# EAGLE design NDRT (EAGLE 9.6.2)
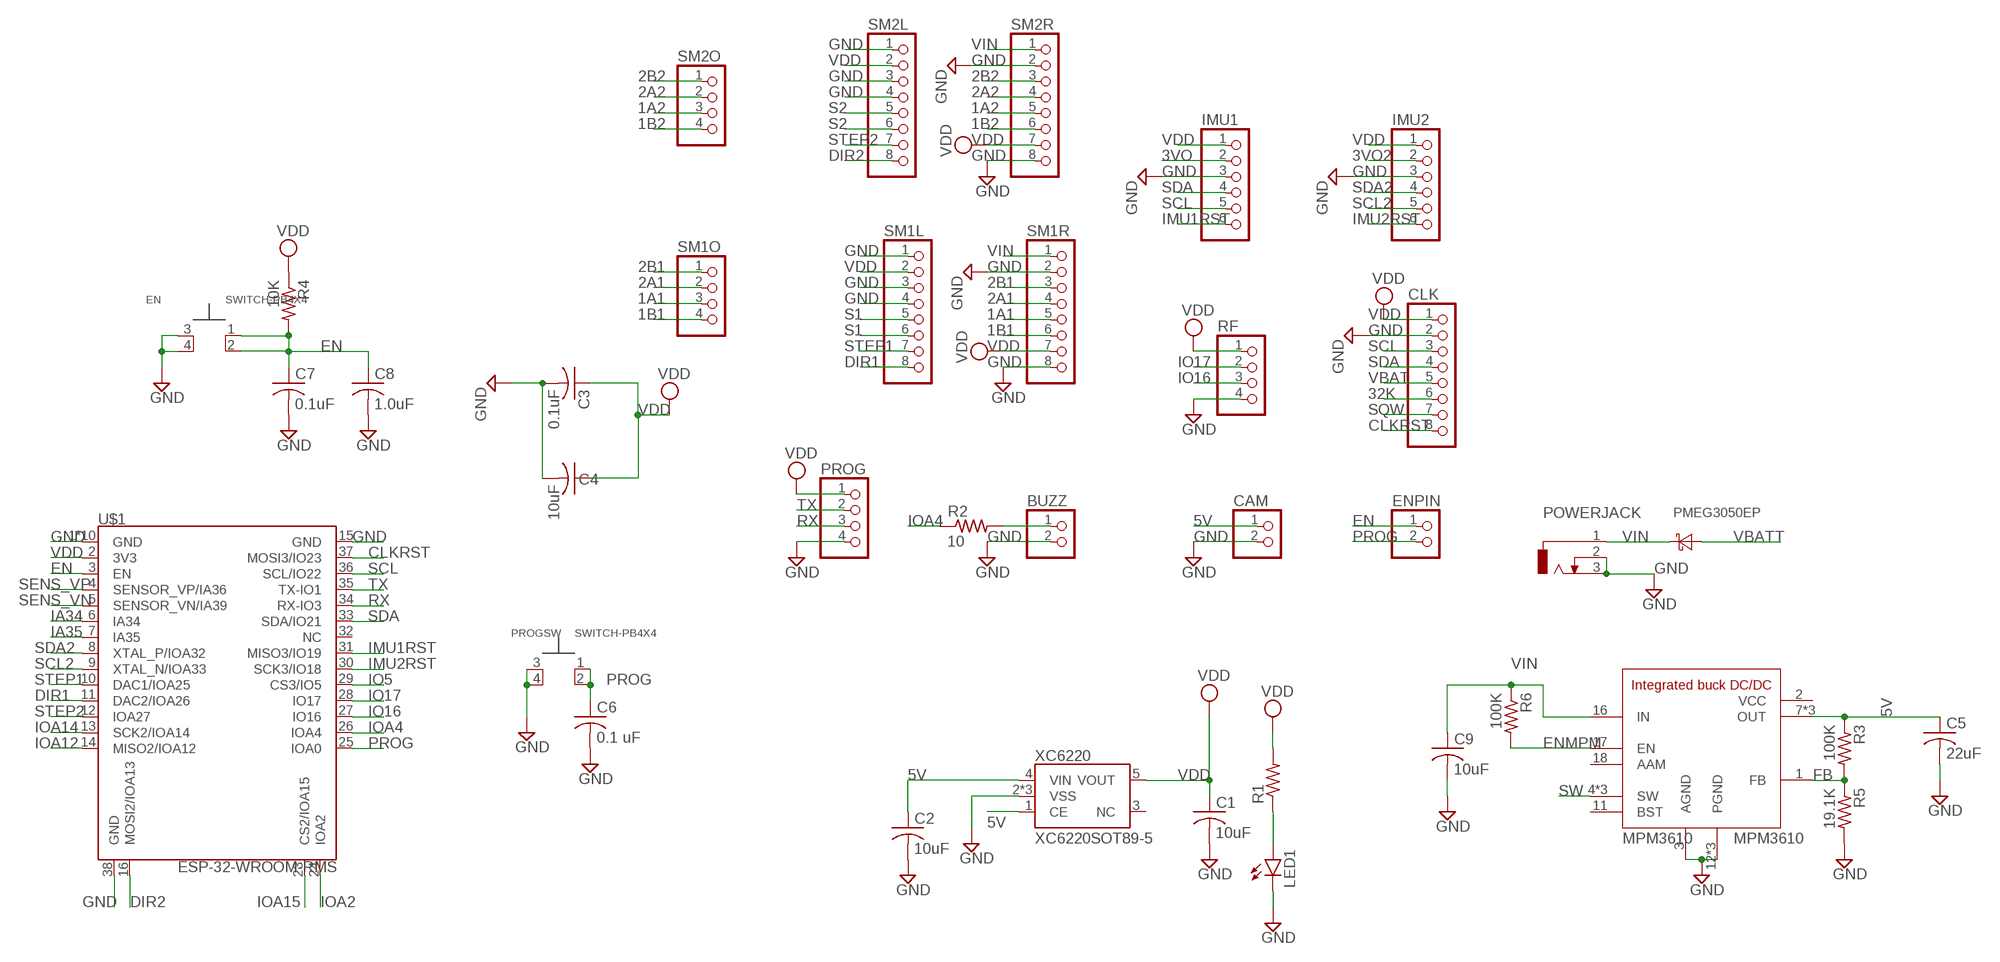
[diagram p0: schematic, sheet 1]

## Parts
BUZZ  PINHD-1X2S  [1X02N]
C1  10uF  C-USC0805  [C0805]
C2  10uF  C-USC0805  [C0805]
C3  0.1uF  C-USC0603  [C0603]
C4  10uF  C-USC0805  [C0805]
C5  22uF  C-USC0805  [C0805]
C6  0.1 uF  C-USC0603  [C0603]
C7  0.1uF  C-USC0603  [C0603]
C8  1.0uF  C-USC0603  [C0603]
C9  10uF  C-USC0805  [C0805]
CAM  PINHD-1X2S  [1X02N]
CLK  PINHD-1X8  [1X08]
EN  SWITCH-PB4X4  [PBSMT4X4M]
ENPIN  PINHD-1X2S  [1X02N]
IMU1  PINHD-1X6  [1X06]
IMU2  PINHD-1X6  [1X06]
LED1  LEDCHIPLED_0603  [CHIPLED_0603]
MPM3610  MICROBUILDER_MPM3610  [MICROBUILDER_MPM3610]
PMEG3050EP  DIODE-SCHOTTKY-SOD128  [SOD128]
POWERJACK  DCJ0303  [DCJ0303]
PROG  PINHD-1X4  [1X04N]
PROGSW  SWITCH-PB4X4  [PBSMT4X4M]
R1  R-US_R0603  [R0603]
R2  10  R-US_R0603  [R0603]
R3  100K  R-US_R0603  [R0603]
R4  10K  R-US_R0603  [R0603]
R5  19.1K  R-US_R0603  [R0603]
R6  100K  R-US_R0603  [R0603]
RF  PINHD-1X4  [1X04N]
SM1L  PINHD-1X8  [1X08]
SM1O  PINHD-1X4  [1X04N]
SM1R  PINHD-1X8  [1X08]
SM2L  PINHD-1X8  [1X08]
SM2O  PINHD-1X4  [1X04N]
SM2R  PINHD-1X8  [1X08]
U$1  ESP-32-WROOM-RMS  [ESP-WROOM-32D]
XC6220  XC6220SOT89-5  [SOT89-5]

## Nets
1A1: SM1O.3 SM1R.5
1A2: SM2O.3 SM2R.5
1B1: SM1O.4 SM1R.6
1B2: SM2O.4 SM2R.6
2A1: SM1O.2 SM1R.4
2A2: SM2O.2 SM2R.4
2B1: SM1O.1 SM1R.3
2B2: SM2O.1 SM2R.3
3VO [not power]: IMU1.2
3VO2 [not power]: IMU2.2
5V: C2.1 C5.1 CAM.1 MPM3610.7(OUT) MPM3610.8(OUT) MPM3610.9(OUT) R3.1 XC6220.1(CE) XC6220.4(VIN)
32K [not power]: CLK.6
CLKRST: CLK.8 U$1.37(MOSI3/IO23)
DIR1: SM1L.8 U$1.11(DAC2/IOA26)
DIR2: SM2L.8 U$1.16(MOSI2/IOA13)
EN: C7.1 C8.1 EN.1 EN.2 ENPIN.1 R4.2 U$1.3(EN)
ENMPM: MPM3610.17(EN) R6.2
FB: MPM3610.1(FB) R3.2 R5.1
GND: BUZZ.2 C1.2 C2.2 C3.2 C4.2 C5.2 C6.2 C7.2 C8.2 C9.2 CAM.2 CLK.2 EN.3 EN.4 IMU1.3 IMU2.3 LED1.C MPM3610.3(AGND) MPM3610.12(PGND) MPM3610.13(PGND) MPM3610.14(PGND) POWERJACK.2 POWERJACK.3 PROG.4 PROGSW.3 PROGSW.4 R5.2 RF.4 SM1L.1 SM1L.3 SM1L.4 SM1R.2 SM1R.8 SM2L.1 SM2L.3 SM2L.4 SM2R.2 SM2R.8 U$1.1(GND) U$1.15(GND) U$1.38(GND) U$1.GND U$1.GNDT1(GND) U$1.GNDT2(GND) U$1.GNDT3(GND) U$1.GNDT4(GND) U$1.GNDT5(GND) U$1.GNDT6(GND) U$1.GNDT7(GND) U$1.GNDT8(GND) XC6220.2(VSS) XC6220.6(VSS) XC6220.7(VSS)
IA34 [not power]: U$1.6(IA34)
IA35 [not power]: U$1.7(IA35)
IMU1RST: IMU1.6 U$1.31(MISO3/IO19)
IMU2RST: IMU2.6 U$1.30(SCK3/IO18)
IO5 [not power]: U$1.29(CS3/IO5)
IO16: RF.3 U$1.27(IO16)
IO17: RF.2 U$1.28(IO17)
IOA2 [not power]: U$1.24(IOA2)
IOA4: R2.1 U$1.26(IOA4)
IOA12 [not power]: U$1.14(MISO2/IOA12)
IOA14 [not power]: U$1.13(SCK2/IOA14)
IOA15 [not power]: U$1.23(CS2/IOA15)
N$1: BUZZ.1 R2.2
N$2: LED1.A R1.1
PROG: C6.1 ENPIN.2 PROGSW.1 PROGSW.2 U$1.25(IOA0)
RX: PROG.3 U$1.34(RX-IO3)
S1: SM1L.5 SM1L.6
S2: SM2L.5 SM2L.6
SCL: CLK.3 IMU1.5 U$1.36(SCL/IO22)
SCL2: IMU2.5 U$1.9(XTAL_N/IOA33)
SDA: CLK.4 IMU1.4 U$1.33(SDA/IO21)
SDA2: IMU2.4 U$1.8(XTAL_P/IOA32)
SENS_VN [not power]: U$1.5(SENSOR_VN/IA39)
SENS_VP [not power]: U$1.4(SENSOR_VP/IA36)
SQW [not power]: CLK.7
STEP1: SM1L.7 U$1.10(DAC1/IOA25)
STEP2: SM2L.7 U$1.12(IOA27)
SW: MPM3610.4(SW) MPM3610.5(SW) MPM3610.6(SW)
TX: PROG.2 U$1.35(TX-IO1)
VBAT [not power]: CLK.5
VBATT: PMEG3050EP.A
VDD: C1.1 C3.1 C4.1 CLK.1 IMU1.1 IMU2.1 PROG.1 R1.2 R4.1 RF.1 SM1L.2 SM1R.7 SM2L.2 SM2R.7 U$1.2(3V3) XC6220.5(VOUT)
VIN: C9.1 MPM3610.16(IN) PMEG3050EP.C POWERJACK.1 R6.1 SM1R.1 SM2R.1
Unconnected: MPM3610.11(BST) MPM3610.18(AAM) U$1.32(NC) XC6220.3(NC)

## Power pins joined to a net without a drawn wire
VCC: MPM3610.2(VCC)

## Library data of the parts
BUZZ CAM ENPIN = newSDlib:PINHD-1X2S: PIN HEADER
C1-C9 = rcl:C-US: CAPACITOR, American symbol; SPICEPREFIX: C
CLK SM1L SM1R SM2L SM2R = pinhead:PINHD-1X8: PIN HEADER
EN PROGSW = newSDlib:SWITCH-PB
IMU1 IMU2 = pinhead:PINHD-1X6: PIN HEADER
LED1 = led:LED: LED
MPM3610 = NDRT:MICROBUILDER_MPM3610
PMEG3050EP = diode:DIODE-SCHOTTKY-: SCHOTTKY DIODE
POWERJACK = con-jack:DCJ0303: DC POWER JACK Source: DCJ0303.pdf; OC_FARNELL: unknown; OC_NEWARK: unknown
PROG RF SM1O SM2O = newSDlib:PINHD-1X4: PIN HEADER
R1-R6 = rcl:R-US_: RESISTOR, American symbol; SPICEPREFIX: R
U$1 = newSDlib:ESP-32-WROOM-RMS
XC6220 = newSDlib:XC6220: Linear Voltage Regulator 1 A max

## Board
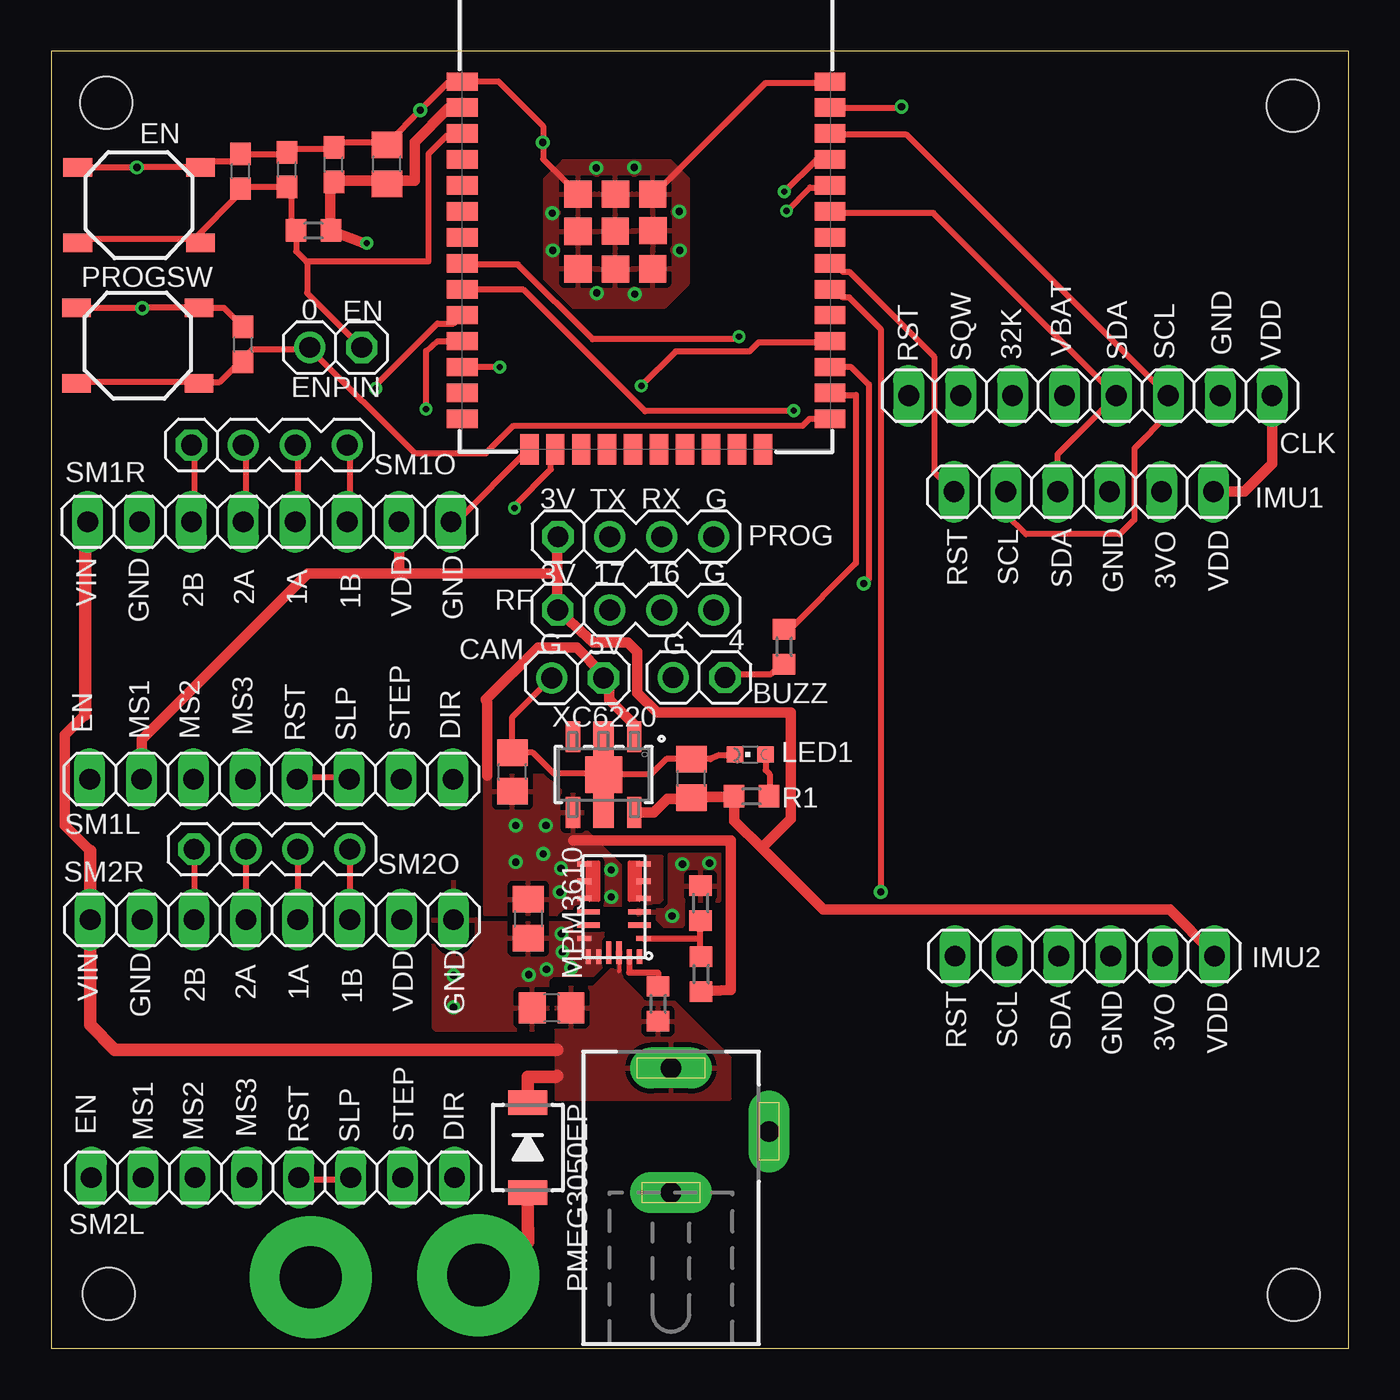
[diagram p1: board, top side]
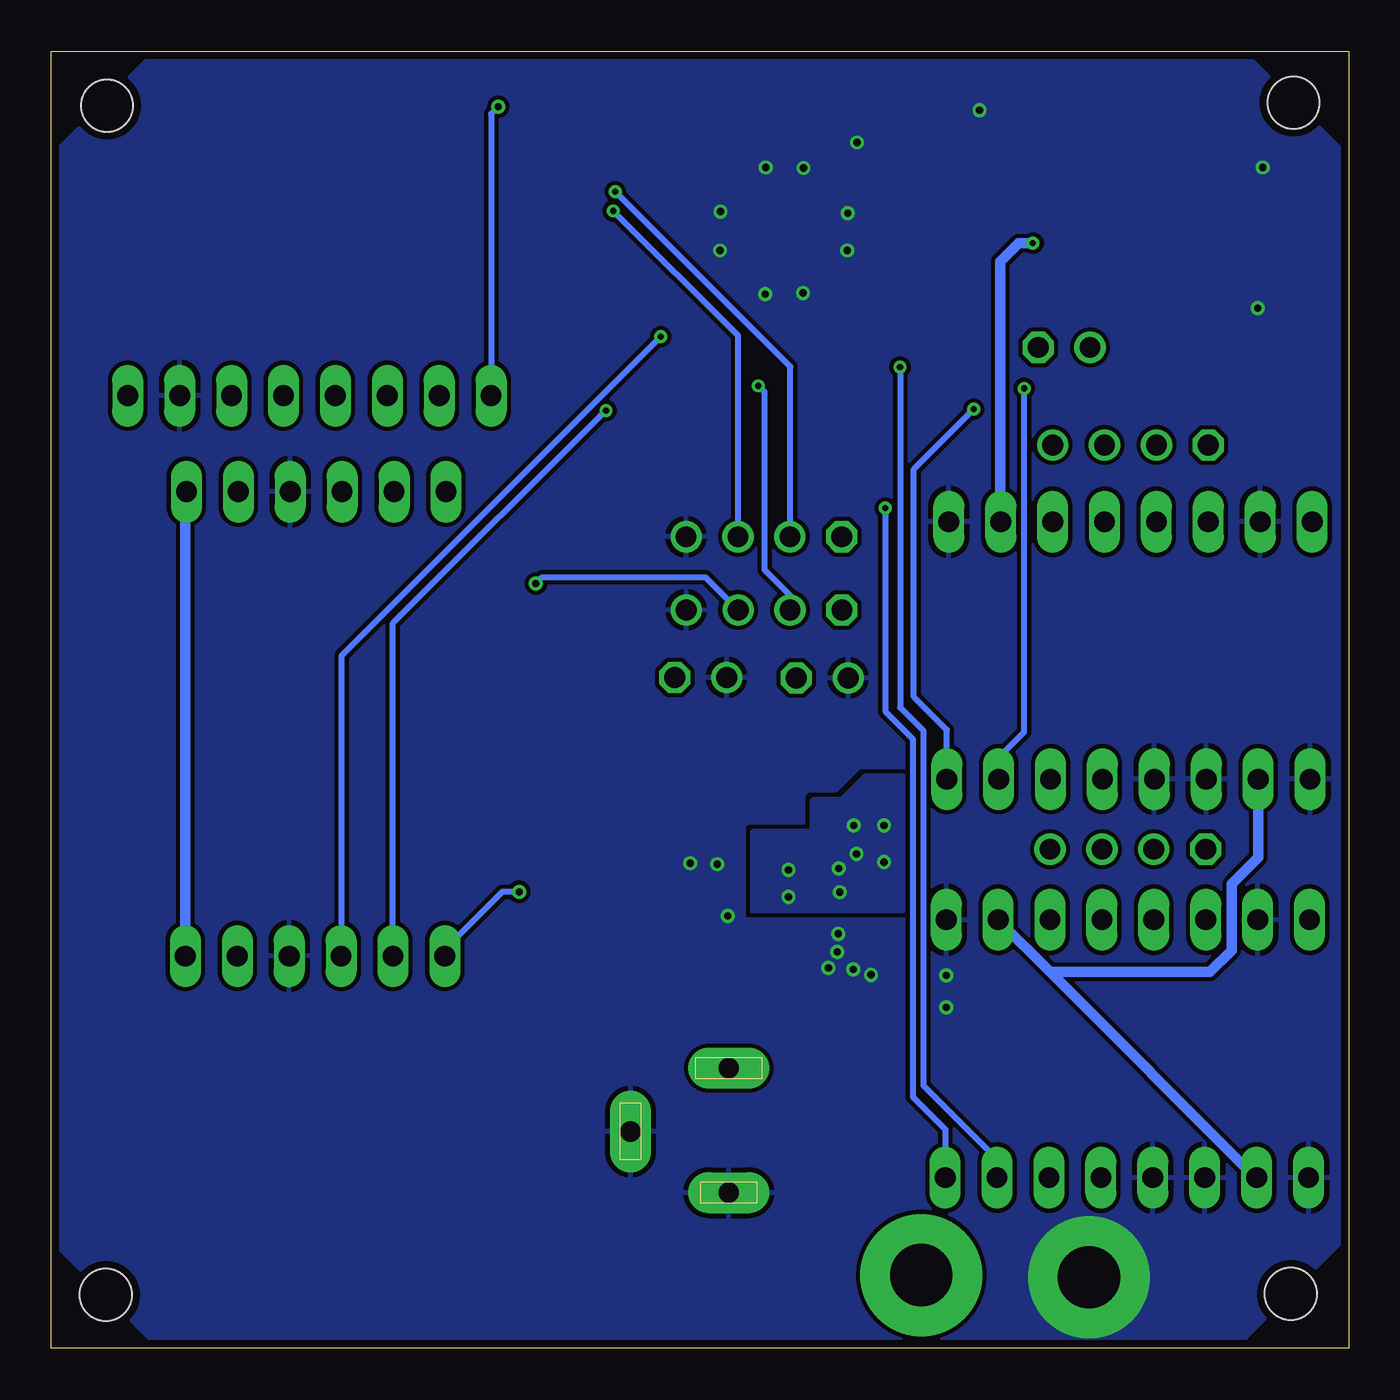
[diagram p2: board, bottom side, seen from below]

Size 63.5 x 63.51 mm. Coordinates in mm from the lower left corner, seen from the top.
Outline: 0,0 63.5,0 63.5,63.51 0.01,63.5 0,0
Copper layers (1*16): Top 0.035559375mm / dielectric 1.6mm / Bottom 0.035559375mm
Design rules "low-cost-2layer": minimum track width 8mil, minimum drill 0.3mm, track to track 8mil, track to pad 8mil, pad to pad 8mil, via to via 8mil, smd to smd 8mil, copper to edge 15mil, drill to drill 8mil, minimum pad ring 6.5mil, minimum via ring 6.5mil, stop-mask expansion 2.5mil, vias tented up to drill 0mil, thermal gap 10mil
Holes 2.54 mm at 2.7,60.99 2.83,2.67 60.82,2.62 60.77,60.84

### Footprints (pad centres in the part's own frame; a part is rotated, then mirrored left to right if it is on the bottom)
1X02N = drill 1.016 octagon: 1 -1.27,0 | drill 1.016: 2 1.27,0
C0805 = smd 1.3 x 1.5: 1 -0.95,0; 2 0.95,0
C0603 = smd 1.1 x 1: 1 -0.85,0; 2 0.85,0
1X08 = drill 1.016 long: 1 -8.89,0; 2 -6.35,0; 3 -3.81,0; 4 -1.27,0; 5 1.27,0; 6 3.81,0; 7 6.35,0; 8 8.89,0
PBSMT4X4M = smd 1.4 x 0.9: 1 -3,1.85; 2 3,1.85; 3 3,-1.85; 4 -3,-1.85
1X06 = drill 1.016 long: 1 -6.35,0; 2 -3.81,0; 3 -1.27,0; 4 1.27,0; 5 3.81,0; 6 6.35,0
CHIPLED_0603 = smd 0.8 x 0.8: A 0,-0.75; C 0,0.75
MICROBUILDER_MPM3610 = smd 0.7 x 0.25: 1 -1.45,1.55; 4 -1.45,-0.4; 5 -1.45,-1.25; 6 -1.45,-2.1; 7 1.45,-2.1; 8 1.45,-1.25; 9 1.45,-0.4; 12 1.45,1.55 | smd 1.1 x 0.25: 2 -1.25,0.9; 3 -1.25,0.25; 10 1.25,0.25; 11 1.25,0.9 | smd 0.25 x 0.7: 13 1.25,2.45; 14 0.75,2.45; 17 -0.75,2.45; 18 -1.25,2.45 | smd 0.25 x 1.1: 15 0.25,2.25; 16 -0.25,2.25
SOD128 = smd 1.2 x 1.9: A 2.2,0; C -2.2,0
DCJ0303 = drill 1 pad 2 long: 1 0,3.1; 2 4.8,0; 3 0,-3
1X04N = drill 1.016 octagon: 1 -3.81,0 | drill 1.016: 2 -1.27,0; 3 1.27,0; 4 3.81,0
R0603 = smd 1 x 1.1: 1 -0.85,0; 2 0.85,0
ESP-WROOM-32D = smd 0.9 x 1.5: 1 7.7,9; 2 6.43,9; 3 5.16,9; 4 3.89,9; 5 2.62,9; 6 1.35,9; 7 0.08,9; 8 -1.19,9; 9 -2.46,9; 10 -3.73,9; 11 -5,9; 12 -6.27,9; 13 -7.54,9; 14 -8.81,9; 25 -8.81,-9; 26 -7.54,-9; 27 -6.27,-9; 28 -5,-9; 29 -3.73,-9; 30 -2.46,-9; 31 -1.19,-9; 32 0.08,-9; 33 1.35,-9; 34 2.62,-9; 35 3.89,-9; 36 5.16,-9; 37 6.43,-9; 38 7.7,-9 | smd 1.5 x 0.9: 15 -10.3,5.715; 16 -10.3,4.445; 17 -10.3,3.175; 18 -10.3,1.905; 19 -10.3,0.635; 20 -10.3,-0.635; 21 -10.3,-1.905; 22 -10.3,-3.175; 23 -10.3,-4.445; 24 -10.3,-5.715 | smd 1.33 x 1.33: GND 0.379,1.515; GNDT1 -1.46,3.33; GNDT2 -1.47,1.5; GNDT3 -1.46,-0.33; GNDT4 0.4,-0.34; GNDT5 2.2,-0.33; GNDT6 2.2,1.5; GNDT7 2.2,3.33; GNDT8 0.37,3.33
SOT89-5 = smd 0.7 x 1.5: 1 -1.5,-1.85; 3 1.5,-1.85; 4 1.5,1.85; 5 -1.5,1.85 | smd 1 x 2: 2 0,-1.6; 6 0,1.6 | smd 1.8 x 1.8: 7 0,0

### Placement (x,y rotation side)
BUZZ  31.71,32.85 180 top
C1  31.34,27.9 90 top
C2  22.58,28.22 90 top
C3  13.84,57.95 90 top
C4  16.44,57.96 90 top
C5  23.35,21.04 270 top
C6  9.4,49.15 90 top
C7  11.55,57.71 90 top
C8  9.28,57.63 90 top
C9  24.5,16.67 180 top
CAM  25.77,32.82 180 top
CLK  50.86,46.64 180 top
EN  4.3,55.97 180 top
ENPIN  13.93,49 180 top
IMU1  50.53,41.94 180 top
IMU2  50.58,19.21 180 top
LED1  34.21,29.08 90 top
MPM3610  27.54,21.62 180 top
PMEG3050EP  23.33,9.84 270 top
POWERJACK  30.34,10.62 0 top
PROG  28.62,39.74 0 top
PROGSW  4.25,49.09 180 top
R1  34.28,27.03 180 top
R2  35.88,34.35 270 top
R3  31.81,18.32 90 top
R4  12.85,54.73 180 top
R5  31.79,21.8 90 top
R6  29.7,16.87 90 top
RF  28.61,36.15 0 top
SM1L  10.78,27.87 0 top
SM1O  10.68,44.23 0 top
SM1R  10.68,40.47 0 top
SM2L  10.86,8.36 0 top
SM2O  10.81,24.44 0 top
SM2R  10.81,20.99 0 top
U$1  29.12,54.31 90 top
XC6220  27.04,28.09 180 top

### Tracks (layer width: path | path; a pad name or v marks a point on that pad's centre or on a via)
1A1
  Top 0.305: SM1R.5 12.08,40.65 12.08,44.14 SM1O.3
1A2
  Top 0.305: SM2O.3 SM2R.5
1B1
  Top 0.305: SM1R.6 14.62,40.65 14.62,44.14 SM1O.4
1B2
  Top 0.305: SM2O.4 SM2R.6
2A1
  Top 0.305: SM1R.4 9.54,40.65 9.54,44.14 SM1O.2
2A2
  Top 0.305: SM2O.2 SM2R.4
2B1
  Top 0.305: SM1R.3 7,40.65 7,44.14 SM1O.1
2B2
  Top 0.305: SM2O.1 SM2R.3
5V  (via drill 0.35)
  Top 0.508: 25.55,24.86 33.27,24.86 33.27,17.54 R3.1 | 22.55,27.31 C2.1 | 23.39,22.02 C5.1 | 21.35,28.05 21.35,31.6 21.28,31.76 23.84,34.31 25.72,34.31 27,33.03 CAM.1 27.32,32.39 27.32,31.76 28.59,30.49 XC6220.1
  other vias: 22.74,23.81 27.42,23.43 27.42,22.1 24.9,22.33 24.95,23.5 24.09,24.21 24.22,25.61 22.74,25.61
  pour Top: 27.82,21.57 25.03,21.57 24.7,21.24 21.27,21.24 21.24,21.27 21.24,27.97 21.32,28.05 24.14,28.05 25.08,27.11 25.89,27.11 25.99,27.01 25.99,25.51 27.82,23.68
  pour Bottom: 21.8,21.39 29.19,21.39 29.19,25.3 29.14,25.36 26.32,25.36 26.27,25.41 26.27,26.83 26.17,26.93 24.8,26.93 23.66,28.07 21.8,28.07
CLKRST  (via drill 0.35)
  Top 0.305: U$1.37 41.57,60.74 v41.62,60.79
  Bottom 0.305: v41.62,60.79 41.97,60.43 CLK.8
DIR1  (via drill 0.3)
  Top 0.305: v18.35,45.98 18.35,48.82 18.91,49.31 U$1.11
  Bottom 0.305: v18.35,45.98 21.28,43.05 21.28,31.9 19.67,30.28 SM1L.8
DIR2  (via drill 0.3)
  Top 0.305: v22.68,41.14 22.68,41.27 24.46,43.05 24.46,43.82 U$1.16
  Bottom 0.305: SM2L.8 19.73,8.38 19.73,10.71 21.33,12.31 21.33,29.83 22.68,31.18 v22.68,41.14
EN
  Top 0.305: 7,54.3 1.6,54.3 EN.2 | 7,54.3 9.22,56.52 C8.1 9.54,56.84 11.44,56.84 C7.1 11.76,56.84 11.76,54.93 R4.2 12,53.71 12.48,53.22 | 7,54.3 EN.1 | ENPIN.1 12.53,51.67 12.53,53.17 12.48,53.22 | 12.48,53.22 18.48,53.22 18.48,58.48 19.39,59.39 20.03,59.39 U$1.3
ENMPM
  Top 0.305: MPM3610.17 28.29,18.4 29.7,18.4 R6.2
FB
  Top 0.305: 31.76,20.07 31.76,19.31 R3.2 | 31.76,20.07 31.76,20.64 R5.1 | MPM3610.1 31.76,20.07
GND  (via drill 0.35, 3.05 pad 5.97)
  Top 0.305: PROGSW.3 4.45,50.94 | 4.45,50.94 v4.46,50.93 | 4.45,50.94 PROGSW.4 8.46,50.94 C6.2 | EN.3 v4.2,57.82 v4.21,57.82 EN.4 7.31,58.11 8.9,58.11 9.22,58.43 C8.2 9.54,58.43 11.44,58.43 C7.2 11.76,58.74 13.66,58.74 C3.2 13.98,59.06 16.2,59.06 C4.2 16.52,59.06 v18.07,60.61 19.42,61.96 20.06,61.96 U$1.1 21.9,62.01 24.08,59.84 24.08,59.04 | U$1.38 38.11,61.96 34.97,61.96 29.54,56.52 U$1.GNDT5 | LED1.C 33.45,29.05 32.72,29.05 32.26,28.85 C1.2 30.1,28.85 29.33,28.09 XC6220.7 | 27.03,28.14 24.6,28.14 23.57,29.17 C2.2 22.58,30.92 24.48,32.82 CAM.2 | XC6220.7 XC6220.6 | XC6220.2 27.05,28.26 27,28.26 27.03,28.14 | 27.03,28.14 XC6220.7 | 23.51,20.01 C5.2 | U$1.15 23.19,43.82 20.01,40.65 19.7,40.65 SM1R.8 | U$1.GNDT7 24.08,58.22 24.08,59.04 | 24.08,59.04 v24.06,59.04
  other vias: 12.71,3.49 25.03,19.41 24.98,20.3 19.7,16.69 19.7,18.27 30.39,21.16 30.9,23.7 32.22,23.76 25.46,18.62 24.24,18.55 23.38,18.29 24.52,55.58 24.55,53.75 26.71,51.67 28.56,51.62 30.77,53.75 30.74,55.66 28.53,57.82 26.68,57.79
  pour Bottom (rank 2): 4.76,63.15 58.79,63.15 63.13,58.81 63.13,4.88 58.73,0.49 5.01,0.49 0.44,5.06 0.44,58.83
  pour Top: 24.17,57.21 24.17,52.18 25.33,51.01 30.03,51.01 31.18,52.15 31.18,57.23 30.31,58.1 25.05,58.1
  pour Top: 25.99,20.22 26.78,20.22 26.96,20.05 26.96,18.73 26.5,18.27 24.52,18.27 24.29,18.04 24.29,15.6 18.83,15.6 18.73,15.7 18.73,22.84 20.66,22.84 20.76,22.74 20.76,20.83 25.38,20.83
  pour Top: 28.71,21.47 30.03,21.47 30.29,21.72 30.29,24.19 32.7,24.19 32.7,21.95 32.65,21.9 30.95,21.9 30.92,21.93 30.92,20.73 30.85,20.66 30.03,20.66 29.45,21.24 28.71,21.24
  pour Top (no thermals): 27.01,20.38 25.28,20.38 25.28,18.6 25.51,18.37 26.65,18.37 27.01,18.73
IMU1RST
  Top 0.305: U$1.31 38.43,53.03 38.75,52.71 39.06,52.71 43.22,48.56 43.22,42.91 IMU1.6
IMU2RST  (via drill 0.35)
  Top 0.305: v40.6,22.36 40.6,49.9 39.06,51.44 38.75,51.44 38.43,51.76 U$1.30
  Bottom 0.305: v40.6,22.36 41.41,22.36 44.23,19.54 IMU2.6
IO16  (via drill 0.35)
  Top 0.305: U$1.27 38.13,48.04 39.16,48.04 40.02,47.19 40.02,37.68 v39.78,37.45
  Bottom 0.305: RF.3 31.48,37.75 39.47,37.75 v39.78,37.45
IO17  (via drill 0.3)
  Top 0.305: v28.89,47.12 30.57,48.8 34.17,48.8 34.63,49.26 38.11,49.26 U$1.28
  Bottom 0.305: v28.89,47.12 28.59,46.82 28.59,38.11 27.32,36.84 27.32,36.2 RF.2
IOA4
  Top 0.305: U$1.26 38.43,46.68 39.38,46.68 39.38,38.44 36.14,35.2 R2.1
N$1
  Top 0.305: R2.2 35.57,33.34 35.25,33.03 33.03,33.03 BUZZ.1
N$2
  Top 0.305: LED1.A 34.96,28.32 35.16,28.12 35.16,27.06 R1.1
PROG
  Top 0.305: PROGSW.2 1.28,47.31 7,47.31 PROGSW.1 7.31,47.31 8.27,47.31 9.22,48.27 C6.1 9.54,48.58 9.85,48.9 12.39,48.9 ENPIN.2 12.71,48.9 17.79,43.82 21.28,43.82 22.63,45.17 36.78,45.17 37.11,45.5 U$1.25
RX  (via drill 0.3)
  Top 0.305: v35.99,55.68 37.13,56.83 38.1,56.83 38.11,56.84 U$1.34
  Bottom 0.305: v35.99,55.68 29.89,49.58 PROG.3
S1
  Top 0.305: SM1L.5 12.08,27.95 14.3,27.95 SM1L.6
S2
  Top 0.305: SM2L.5 12.39,8.26 14.62,8.26 SM2L.6
SCL
  Top 0.305: U$1.36 38.3,59.42 41.88,59.42 54.62,46.68 CLK.3 54.67,45.74 54.68,45.74 53.01,44.06 53.01,40.57 52.3,39.86 47.71,39.86 46.72,40.85 IMU1.5
SCL2  (via drill 0.3)
  Top 0.305: v36.35,45.9 36.35,45.88 29.07,45.88 23.12,51.82 20.19,51.82 U$1.9
  Bottom 0.305: v36.35,45.9 36.35,45.93 46.77,35.5 IMU2.5
SDA
  Top 0.305: U$1.33 38.39,55.58 43.18,55.58 52.08,46.68 CLK.4 49.26,43.77 IMU1.4
SDA2  (via drill 0.3)
  Top 0.305: v33.67,49.54 33.54,49.41 26.5,49.41 22.85,53.07 20.24,53.07 U$1.8
  Bottom 0.305: v33.67,49.54 49.29,33.92 49.29,19.32 49.31,19.29 IMU2.4
STEP1  (via drill 0.3)
  Top 0.305: v15.89,47 15.89,47.15 18.91,50.17 19.7,50.17 20.01,50.49 U$1.10
  Bottom 0.305: v15.89,47 15.89,30.17 17.12,28.94 17.12,27.87 SM1L.7
STEP2  (via drill 0.3)
  Top 0.305: v21.96,48.04 U$1.12
  Bottom 0.305: SM2L.7 17.47,8.58 17.47,9.53 20.82,12.88 20.82,30.24 21.96,31.38 v21.96,48.04
SW
  pour Top (rank 2, no thermals): 28.08,23.91 28.08,21.75 29.91,21.75 29.91,24.06 28.23,24.06
TX  (via drill 0.3)
  Top 0.305: v35.89,56.62 37.44,58.17 38.12,58.17 U$1.35
  Bottom 0.305: v35.89,56.62 27.33,48.06 27.33,40.27 27.35,40.25 PROG.2
VBATT  (via drill 3.05 pad 5.97)
  Top 0.61: PMEG3050EP.A 23.33,5.85 23.35,5.82 23.35,5.21 v20.91,3.59
VDD  (via drill 0.3)
  Top 0.508: XC6220.5 29.48,26.24 30.15,26.91 31.3,26.91 C1.1 31.44,26.99 33.35,26.99 R1.2 33.43,25.83 34.77,24.49 | 34.77,24.49 37.78,21.48 54.73,21.48 56.84,19.37 IMU2.1 | U$1.2 20.06,60.69 19.42,60.69 17.79,59.06 17.79,57.16 16.52,57.16 C4.1 16.2,57.16 13.98,57.16 C3.1 13.66,56.84 13.66,54.93 R4.1 15.31,54.1 v15.45,54.11 | 24.78,37.94 24.78,39.69 PROG.1 | 24.78,37.94 24.78,36.2 RF.1 26.54,34.56 28.22,34.56 28.69,34.09 28.69,32.09 29.65,31.12 36.21,31.12 36.21,25.93 34.77,24.49 | 17.03,37.94 12.56,37.94 4.43,29.81 SM1L.2 | 17.03,37.94 24.78,37.94 | CLK.1 59.75,43.31 58.38,41.94 IMU1.1 | SM1R.7 17.03,37.94
  Bottom 0.508: 14.62,18.42 17.16,20.96 SM2R.7 | 14.62,18.42 4.77,8.58 SM2L.2 | v15.45,54.11 16.14,54.11 17.04,53.21 17.04,40.6 17.03,40.58 SM1R.7 | IMU2.1 56.93,41.89 IMU1.1 | SM1L.2 4.43,24.04 5.73,22.75 5.73,19.49 6.79,18.42 14.62,18.42
VIN
  Top 0.203: MPM3610.16 27.79,18.48
  Top 0.508: 1.92,24.36 0.66,25.61 0.66,30.03 1.67,31.05
  Top 0.61: 1.67,31.05 1.67,40.38 SM1R.1 | 1.92,24.36 SM2R.1 1.92,15.83 3.12,14.62 23.86,14.62 24.14,14.61 24.78,14.61 | PMEG3050EP.C 23.33,13.29 24.7,13.29 24.78,13.34
  pour Top: 27.65,19.41 27.65,18.78 26.53,17.66 24.72,17.66 24.72,12.22 33.21,12.22 33.21,14.23 30.52,16.92 29.09,16.92 27.92,18.09 27.92,19.41 27.9,19.44 27.67,19.44

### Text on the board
tNames: 0 | EN | VBAT | GND | RST | SQW | 32K | SDA | SCL | VDD | 3V | TX | RX | G | 3V | 17 | 16 | G | RST | SCL | SDA | GND | 3VO | VDD | VIN | GND | 2B | 2A | 1A | 1B | VDD | GND | G | 5V | G | 4 | EN | MS1 | MS2 | MS3 | RST | SLP | STEP | DIR | VIN | 2B | 2A | 1A | 1B | GND | VDD | GND | RST | SCL | SDA | 3VO | GND | VDD | EN | MS1 | MS2 | MS3 | RST | SLP | STEP | DIR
